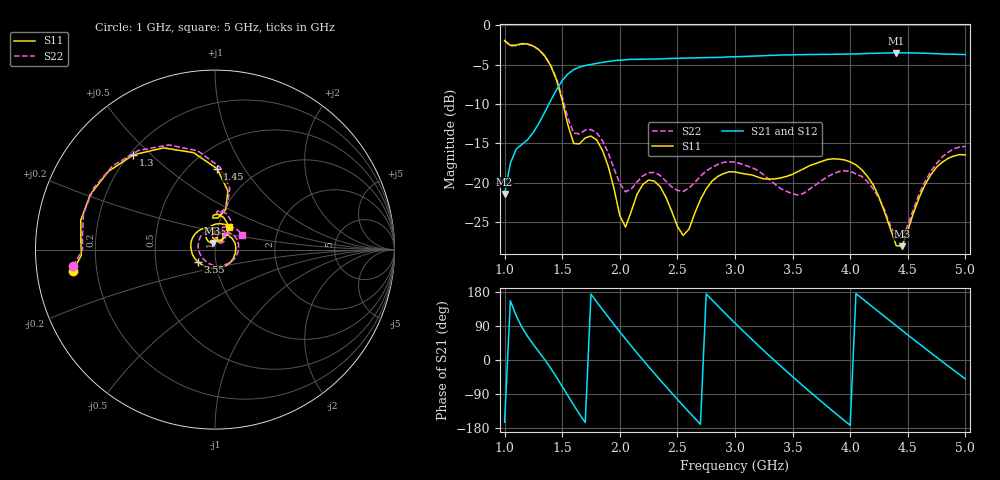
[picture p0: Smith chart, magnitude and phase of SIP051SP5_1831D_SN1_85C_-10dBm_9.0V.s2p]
# GHz  S  dB  R  50
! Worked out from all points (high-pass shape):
!   81 points, 1 GHz to 5 GHz, reference 50 ohm
!   highest |S21| = -3.51 dB at 4.4 GHz (marker M1); lowest = -21.5 dB at 1 GHz (marker M2)
!   |S21| within 3 dB of the highest: 1.531 GHz to end of sweep
!   lowest |S11| = -28.1 dB at 4.45 GHz (marker M3), VSWR 1.08, Z = 48.5 + j3.58 ohm
!   |S11| at or under -10 dB: 1.508 GHz to end of sweep
!   |S22| runs from -27.1 to -2.0 dB; largest |S21 - S12| = 0.0022
!   S11 on the Smith chart (normalised r, x): 1 GHz: 0.11, -0.07; 1.3 GHz: 0.22, +0.44; 1.45 GHz: 0.68, +0.76; 3.55 GHz: 0.82, -0.11; 5 GHz: 1.13, +0.30
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1  -1.93 -171.3  -21.45 -164.1  -21.47 -164.3  -1.98 -173.4
1.3  -3.14 130.7  -12.40 20.7  -12.38 20.9  -3.13 127.6
1.45  -6.93 88.4  -8.21 -44.9  -8.17 -44.9  -6.76 86.4
1.55  -12.71 75.1  -6.18 -94.4  -6.17 -94.4  -11.85 74.5
1.7  -14.33 93.0  -5.12 -164.9  -5.11 -164.9  -13.33 86.2
1.85  -15.91 64.4  -4.72 133.0  -4.71 133.0  -14.68 61.8
2  -24.19 59.1  -4.43 74.5  -4.41 74.5  -20.09 56.3
2.2  -20.23 92.9  -4.31 0.3  -4.31 0.3  -19.14 74.4
2.35  -20.52 63.3  -4.27 -52.6  -4.25 -52.5  -19.09 58.5
2.5  -25.57 53.7  -4.21 -103.8  -4.20 -103.9  -20.99 54.5
2.7  -22.16 78.4  -4.12 -169.7  -4.11 -169.6  -19.19 57.3
2.85  -19.22 46.3  -4.09 143.1  -4.07 143.0  -17.70 38.8
3  -18.65 4.7  -4.01 97.4  -3.99 97.5  -17.42 13.1
3.3  -19.56 -83.8  -3.83 10.8  -3.83 10.8  -19.66 -51.5
3.55  -18.58 -145.3  -3.74 -57.4  -3.73 -57.5  -21.58 -137.0
3.7  -17.59 -177.6  -3.71 -96.8  -3.70 -96.8  -20.30 167.3
4.05  -17.75 111.8  -3.65 175.3  -3.62 175.2  -18.89 76.7
4.35  -25.93 79.5  -3.51 102.3  -3.53 102.3  -25.52 44.4
4.4  -28.04 90.5  -3.51 90.3  -3.50 90.3  -26.91 52.5
4.45  -28.09 110.7  -3.51 78.3  -3.50 78.3  -27.09 70.0
4.75  -18.04 106.1  -3.61 7.3  -3.61 7.3  -17.59 69.9
5  -16.49 59.1  -3.72 -50.0  -3.72 -50.0  -15.40 29.1
